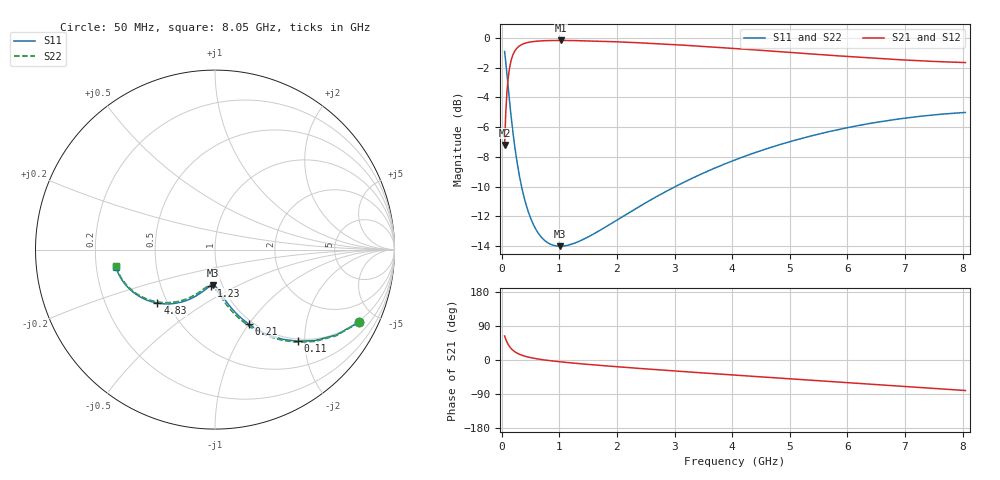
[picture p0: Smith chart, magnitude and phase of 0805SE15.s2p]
! AVX Thin Film Operation		Date: August 2001
! Description: Accu-P® Series, Thin Film, SMD, RF Capacitor
! Part Number: 08055J150FBT
! 50 MHz  -  8.05 GHz
! Serial Measurements
# mhz S db R 50
!	S11		S21		S12		S22
!	dB	Phase	dB	Phase	dB	Phase	dB	Phase
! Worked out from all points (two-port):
!   401 points, 50 MHz to 8.05 GHz, reference 50 ohm
!   highest |S21| = -0.18 dB at 1.03 GHz (marker M1); lowest = -7.2 dB at 50 MHz (marker M2)
!   |S21| within 3 dB of the highest: 101.1 MHz to end of sweep
!   lowest |S11| = -14.0 dB at 1.01 GHz (marker M3), VSWR 1.50, Z = 45.3 - j18.8 ohm
!   |S11| at or under -10 dB: 344.5 MHz to 3.015 GHz (2.67 GHz wide, 159 % of centre)
!   |S22| runs from -14.0 to -0.9 dB; largest |S21 - S12| = 0
!   S11 on the Smith chart (normalised r, x): 50 MHz: 0.96, -4.03; 110 MHz: 0.95, -1.85; 210 MHz: 0.95, -1.00; 1.23 GHz: 0.88, -0.37; 4.83 GHz: 0.44, -0.33; 8.05 GHz: 0.28, -0.08
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50  -0.92 -26.5  -7.20 63.3  -7.20 63.3  -0.92 -26.8
70  -1.64 -35.0  -5.03 54.8  -5.03 54.8  -1.64 -35.4
110  -3.26 -48.0  -2.78 41.6  -2.78 41.6  -3.26 -48.7
150  -4.82 -56.9  -1.74 32.6  -1.74 32.6  -4.82 -57.8
170  -5.54 -60.3  -1.42 29.2  -1.42 29.2  -5.54 -61.3
210  -6.84 -65.7  -1.01 23.7  -1.01 23.7  -6.84 -66.9
270  -8.45 -71.3  -0.67 17.9  -0.67 17.9  -8.45 -72.9
330  -9.73 -75.3  -0.49 13.7  -0.49 13.7  -9.73 -77.1
430  -11.31 -80.0  -0.34 8.9  -0.34 8.9  -11.31 -82.2
530  -12.39 -83.3  -0.26 5.4  -0.26 5.4  -12.39 -85.8
750  -13.64 -88.5  -0.20 -0.1  -0.20 -0.1  -13.64 -91.4
1010  -14.01 -93.1  -0.18 -4.7  -0.18 -4.7  -14.01 -96.2
1030  -14.01 -93.4  -0.18 -5.0  -0.18 -5.0  -14.01 -96.5
1230  -13.85 -96.4  -0.19 -8.0  -0.19 -8.0  -13.85 -99.4
1390  -13.60 -98.6  -0.20 -10.2  -0.20 -10.2  -13.60 -101.6
2010  -12.23 -106.5  -0.27 -17.9  -0.27 -17.9  -12.23 -109.0
2730  -10.59 -114.8  -0.40 -26.0  -0.40 -26.0  -10.59 -116.9
4050  -8.21 -129.0  -0.72 -39.9  -0.72 -39.9  -8.21 -130.6
4830  -7.18 -137.1  -0.93 -47.9  -0.93 -47.9  -7.18 -138.4
5390  -6.58 -142.8  -1.09 -53.5  -1.09 -53.5  -6.58 -144.0
6730  -5.55 -156.3  -1.44 -67.0  -1.44 -67.0  -5.55 -157.4
8050  -5.02 -169.8  -1.66 -80.5  -1.66 -80.5  -5.02 -170.9
